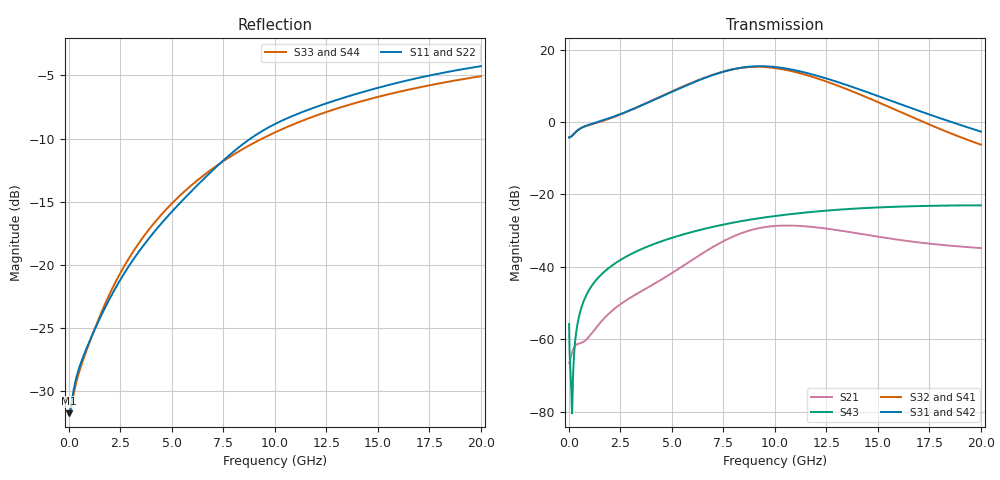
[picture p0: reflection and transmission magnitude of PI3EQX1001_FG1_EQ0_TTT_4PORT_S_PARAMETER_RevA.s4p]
! NPort=4 DATA=2000 NOISE=0 GROUPDELAY=0 COMPLEX_DATAFORMAT=POLAR
! NumOfBlock=1 NumOfParam=0
! .MODEL Smodel S TSTONEFILE=PI3EQX1001_FG1_EQ0_TTT_4PORT_S_PARAMETER_RevA.s4p TYPE=S
!  -- The above .MODEL line can be used for the S element in the netlist.
! The s parameter is extracted from the linear redriver, it is not bi-directional; only s(4,1)s(4,2) and s(3,1)s(3,2)
! should be the insertion loss
!Port definition:
!Port1 = input+
!Port2 = input¨C
!Port3 = output+
!Port4 = output-
# Hz S MA R  50
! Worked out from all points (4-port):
!   2000 points, 10 MHz to 20 GHz, reference 50 ohm
!   strongest paths, dB at 10 MHz, 5.01 GHz, 10.01 GHz, 15.01 GHz, 20 GHz:
!     S31: -4.3, 8.3, 15.2, 7.1, -2.7
!     S42: -4.3, 8.3, 15.2, 7.1, -2.7
!     S32: -4.3, 8.5, 14.9, 5.5, -6.3
!     S41: -4.3, 8.5, 14.8, 5.4, -6.3
!     S43: -55.8, -32.0, -26.0, -23.6, -23.0
!     S21: -66.5, -41.7, -28.7, -31.7, -34.8
!   lowest |S11| = -31.7 dB at 10 MHz (marker M1), VSWR 1.05, Z = 47.5 - j0.063 ohm
!   |S11| at or under -10 dB: start of sweep to 8.817 GHz
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1e7  0.02591 -178.5  0.0004939 2.7  3.669e-05 -0.2  4.787e-05 -0.1
     0.0004742 2.9  0.02597 -178.7  4.577e-05 -0.2  5.994e-05 -0.1
     0.612 0.1  0.612 -179.9  0.02616 178.4  0.001614 -59.2
     0.6117 -179.9  0.6118 0.1  0.001627 -58.9  0.02612 178.4
6.34e9  0.2108 -105.0  0.01381 96.9  2.285e-05 -30.8  3.284e-05 -29.3
        0.01451 95.3  0.2092 -105.0  2.995e-05 -26.4  4.148e-05 -24.6
        3.793 -51.5  3.839 131.7  0.2196 -111.3  0.03226 59.6
        3.83 131.7  3.791 -51.3  0.03224 59.6  0.2195 -111.3
8.35e9  0.2964 -106.8  0.0279 69.6  2.034e-05 -28.3  3.182e-05 -31.6
        0.02902 68.1  0.2946 -106.8  2.95e-05 -25.9  3.897e-05 -24.3
        5.608 -110.2  5.568 72.9  0.2845 -113.7  0.04279 47.4
        5.548 73.0  5.609 -110.1  0.04271 47.3  0.2843 -113.6
1.019e10  0.3673 -112.0  0.03572 34.4  2.171e-05 -23.3  3.261e-05 -39.0
          0.037 33.0  0.3647 -112.1  3.087e-05 -32.2  4.017e-05 -23.6
          5.66 -171.7  5.451 11.7  0.3399 -116.5  0.05129 35.5
          5.428 11.9  5.662 -171.5  0.05113 35.5  0.3397 -116.5
1.268e10  0.4407 -117.8  0.03213 -2.0  2.777e-05 -35.8  3.05e-05 -57.4
          0.03323 -3.2  0.437 -117.9  2.896e-05 -48.9  4.53e-05 -33.3
          3.841 116.3  3.469 -59.4  0.4074 -120.5  0.06048 19.7
          3.452 -59.2  3.842 116.4  0.06036 19.8  0.4073 -120.5
1.532e10  0.51 -122.7  0.0244 -21.8  2.771e-05 -66.8  2.325e-05 -84.5
          0.0253 -23.0  0.5056 -122.8  2.15e-05 -72.6  4.267e-05 -54.7
          2.116 57.3  1.718 -115.8  0.4692 -124.7  0.06676 3.5
          1.708 -115.4  2.116 57.4  0.06673 3.6  0.4687 -124.7
2e10  0.6113 -130.9  0.01756 -32.5  1.325e-05 -152.8  1.074e-05 150.7
      0.01818 -34.4  0.6059 -130.9  6.569e-06 132.9  1.598e-05 -93.7
      0.7367 -16.9  0.4865 -173.0  0.5579 -131.2  0.07072 -23.1
      0.4846 -172.1  0.7359 -16.7  0.07071 -23.2  0.5578 -131.1
